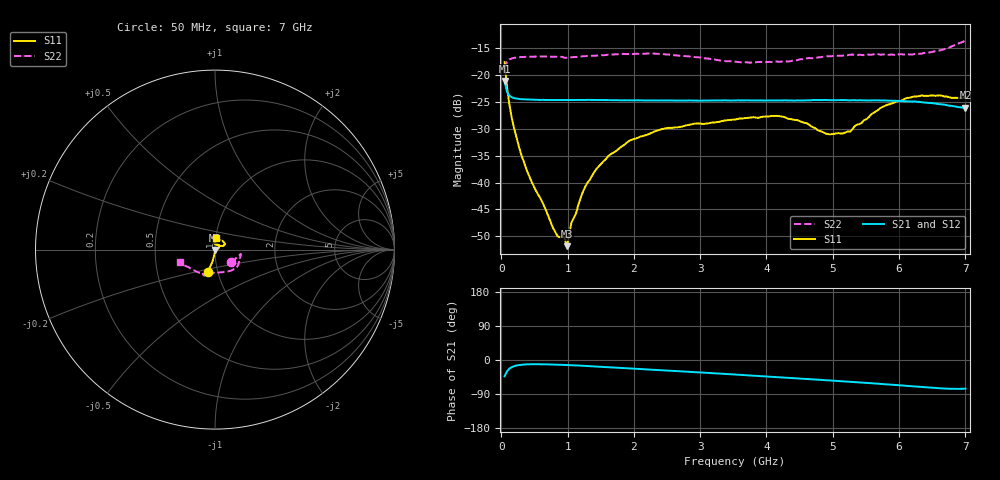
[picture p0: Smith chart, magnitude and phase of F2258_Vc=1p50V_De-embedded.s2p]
! Integrated Device Technology
! Corporate Headquarters
! 6024 Silver Creek Valley Road
! San Jose, CA 95138  USA
! Phone:  1-408-284-8200
! Toll Free:  1-800-223-1366
! Webpage:  http://www.idt.com/
! Timing and RF Division
! 515 Groton Road, Suite 102
! Westford, MA 01886-6024
! Device:  F2258
! Description: Voltage Variable RF Attenuator
! Frequency:  50.0 -  6000.00 MHz
! Package:  3x3 mm Thin QFN Plastic Package: 16 pin
! Ports:  2 RF, 2 DC
!  Pin  1  = NC
!  Pin  2  = NC
!  Pin  3  = RF2  = Port 2
!  Pin  4  = GND
!  Pin  5  = Vdd
!  Pin  6  = NC
!  Pin  7  = VCTRL
!  Pin  8  = NC
!  Pin  9  = GND
!  Pin 10  = RF1  = Port 1
!  Pin 11  = NC
!  Pin 12  = NC
!  Pin 13  = NC
!  Pin 14  = NC
!  Pin 15  = NC
!  Pin 16  = NC
! Vcntrl:  1.500 Volts
! Vdd:  +3.300 Volts
! Current:  1.161 mA
! Data:  The device was measured on a the F2258 evaluation board which has
!  individual transmission lines to the RF pins.  Data was collected
!  using a calibrated network analyzer.  The evaluation board was
!  de-embedded using a TRL calibration technique.
!  The reference plane is the edge of the package pin.
! Misc:  SN 10
!  Action Tracker AT0285
! Date Measured:  2014-12-10
! Date:  2016-01-13  MJV
! Note:
!  Integrated Device Technology supplies this data as a sample of measured
!  data at the package pin for this product.  Your particular data for this
!  product may vary.
!  Data was taken at 25 degrees C.
!  Integrated Device Technology reserves the right to change this data at anytime.
!Freq_(GHz)  S11M_(dB)  S11P_(deg)  S21M_(dB)  S21P_(deg)  S12M_(dB)  S12P_(deg)  S22M_(dB)  S22P_(deg)
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# GHz S dB R 50
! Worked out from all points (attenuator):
!   201 points, 50 MHz to 7 GHz, reference 50 ohm
!   highest |S21| = -21.16 dB at 50 MHz (marker M1); lowest = -26.1 dB at 7 GHz (marker M2)
!   lowest |S11| = -51.8 dB at 988.2 MHz (marker M3), VSWR 1.01, Z = 50.2 - j0.196 ohm
!   |S11| at or under -10 dB: start of sweep to end of sweep
!   |S22| runs from -18.9 to -13.6 dB; largest |S21 - S12| = 0.00048
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0.05  -17.65 -108.2  -21.16 -42.9  -21.12 -42.8  -18.85 -37.9
0.08475  -22.11 -103.2  -23.14 -30.2  -23.11 -30.2  -17.64 -19.0
0.15425  -27.80 -100.2  -24.16 -19.1  -24.11 -19.1  -17.00 -11.7
0.29325  -34.50 -96.7  -24.53 -12.7  -24.48 -12.7  -16.73 -9.8
0.77975  -48.42 -55.6  -24.70 -12.0  -24.65 -12.0  -16.65 -16.3
0.84925  -49.97 -31.4  -24.70 -12.4  -24.65 -12.4  -16.68 -17.6
0.9535  -50.25 -64.0  -24.71 -13.1  -24.67 -13.1  -16.87 -19.2
0.98825  -51.81 -49.5  -24.70 -13.3  -24.67 -13.3  -16.85 -20.2
1.05775  -47.41 -15.0  -24.70 -13.8  -24.66 -13.8  -16.76 -21.3
1.2315  -41.73 7.9  -24.68 -15.2  -24.63 -15.2  -16.57 -24.4
1.44  -37.40 13.2  -24.70 -17.3  -24.64 -17.3  -16.45 -28.0
1.6485  -34.75 17.8  -24.72 -19.3  -24.66 -19.3  -16.28 -31.3
1.9265  -32.29 26.6  -24.75 -22.0  -24.68 -22.0  -16.17 -35.8
2.37825  -30.24 38.1  -24.78 -26.4  -24.75 -26.4  -16.13 -43.0
3.525  -28.31 86.9  -24.77 -38.3  -24.79 -38.3  -17.59 -72.4
4.1505  -27.64 103.2  -24.77 -45.1  -24.78 -45.1  -17.55 -93.9
4.7065  -29.75 93.3  -24.69 -51.2  -24.73 -51.1  -16.92 -105.8
4.94975  -31.07 75.6  -24.72 -53.9  -24.78 -53.8  -16.58 -108.2
5.2625  -30.55 47.0  -24.75 -57.5  -24.75 -57.4  -16.29 -111.1
5.85325  -25.50 25.1  -24.81 -64.8  -24.82 -64.8  -16.30 -115.6
6.33975  -23.83 31.6  -25.11 -71.4  -25.12 -71.4  -16.09 -127.4
7  -24.05 83.6  -26.13 -75.7  -26.12 -75.7  -13.64 -160.1
